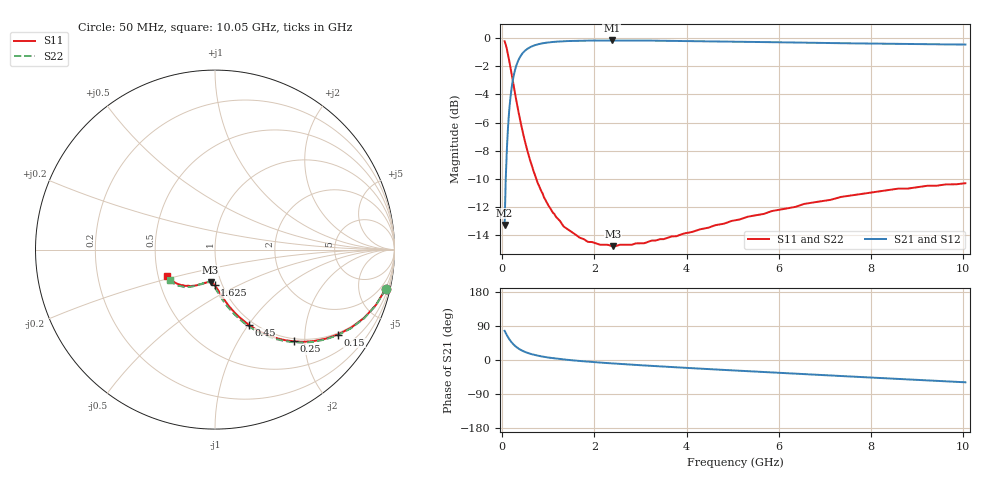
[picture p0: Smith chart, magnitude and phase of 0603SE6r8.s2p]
! AVX Thin Film Operation		Date: August 2001
! Description: Accu-P® Series, Thin Film, SMD, RF Capacitor
! Part Number: 06035J6R8BBT
! 50 MHz  -  10.05 GHz
! Serial Measurements
# mhz S db R 50
!	S11		S21		S12		S22
!	dB	Phase	dB	Phase	dB	Phase	dB	Phase
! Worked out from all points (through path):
!   401 points, 50 MHz to 10.05 GHz, reference 50 ohm
!   highest |S21| = -0.16 dB at 2.375 GHz (marker M1); lowest = -13.3 dB at 50 MHz (marker M2)
!   group delay of S21, straight-line fit = 22.2 ps
!   lowest |S11| = -14.8 dB at 2.4 GHz (marker M3), VSWR 1.44, Z = 44.7 - j16.7 ohm
!   |S11| at or under -10 dB: 736.3 MHz to end of sweep
!   |S22| runs from -14.7 to -0.2 dB; largest |S21 - S12| = 0
!   S11 on the Smith chart (normalised r, x): 50 MHz: 0.95, -8.74; 150 MHz: 0.95, -2.92; 250 MHz: 0.95, -1.77; 450 MHz: 0.95, -1.00; 1.625 GHz: 0.92, -0.38; 10.05 GHz: 0.56, -0.18
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50  -0.21 -12.9  -13.30 77.0  -13.30 77.0  -0.21 -13.0
100  -0.78 -24.7  -7.83 65.2  -7.83 65.2  -0.78 -24.9
125  -1.17 -29.9  -6.27 59.9  -6.27 59.9  -1.17 -30.2
150  -1.60 -34.7  -5.12 55.1  -5.12 55.1  -1.60 -35.1
200  -2.50 -42.8  -3.59 46.9  -3.59 46.9  -2.50 -43.3
250  -3.44 -49.4  -2.62 40.2  -2.62 40.2  -3.44 -50.0
300  -4.36 -54.8  -1.99 34.8  -1.99 34.8  -4.36 -55.5
350  -5.22 -59.2  -1.56 30.4  -1.56 30.4  -5.22 -60.0
450  -6.76 -65.8  -1.03 23.6  -1.03 23.6  -6.76 -66.9
550  -8.07 -70.6  -0.74 18.7  -0.74 18.7  -8.07 -71.9
650  -9.17 -74.2  -0.56 15.0  -0.56 15.0  -9.17 -75.6
950  -11.58 -81.5  -0.32 7.5  -0.32 7.5  -11.58 -83.3
1325  -13.37 -87.1  -0.21 1.5  -0.21 1.5  -13.28 -89.4
1625  -14.06 -90.6  -0.18 -1.9  -0.18 -1.9  -14.06 -92.9
1725  -14.25 -91.7  -0.17 -3.0  -0.17 -3.0  -14.25 -94.0
2375  -14.79 -97.6  -0.16 -8.9  -0.16 -8.9  -14.70 -99.7
2400  -14.80 -97.8  -0.16 -9.1  -0.16 -9.1  -14.70 -99.8
3400  -14.32 -105.8  -0.17 -16.7  -0.17 -16.7  -14.32 -106.8
5050  -12.96 -117.4  -0.24 -27.8  -0.24 -27.8  -12.96 -117.4
6725  -11.70 -129.0  -0.32 -38.3  -0.32 -38.3  -11.70 -127.0
8400  -10.79 -140.2  -0.40 -48.8  -0.40 -48.8  -10.79 -136.2
10050  -10.32 -150.8  -0.45 -58.9  -0.45 -58.9  -10.30 -145.8
